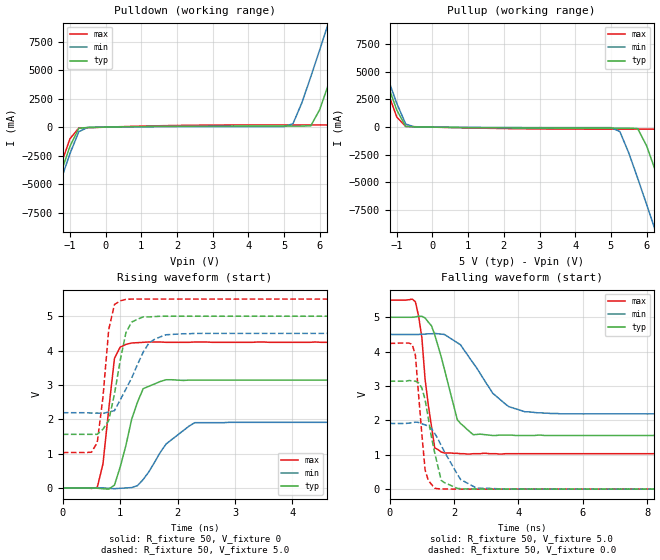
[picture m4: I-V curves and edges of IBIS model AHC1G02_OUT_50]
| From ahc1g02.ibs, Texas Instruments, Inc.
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|   Model AHC1G02_OUT_50
[Model]   AHC1G02_OUT_50
Model_type  Output
Polarity   Inverting
Vmeas = 2.50v
Cref = 15pf
| variable   typ   min   max
C_comp   3.12pf   2.34pf   3.90pf
[Temperature Range]   25   85   -40
[Voltage Range]   5.0   4.5   5.5
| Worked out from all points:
|   slope of the pulldown table from 0 to 0.75 V, typ, clamps not added: 18.8 ohm
|   slope of the pullup table from 0 to 0.75 V, typ, clamps not added: 25.3 ohm
|   rising waveform, R_fixture 50, V_fixture 0: 20-80 % time 302ps typ, 530ps min, 165ps max; typ from 0 V to 3.14 V
|   falling waveform, R_fixture 50, V_fixture 5.0: 20-80 % time 583ps typ, 1.06ns min, 315ps max; typ from 5 V to 1.56 V
|   rising waveform, R_fixture 50, V_fixture 5.0: 20-80 % time 237ps typ, 404ps min, 154ps max; typ from 1.56 V to 5 V
|   falling waveform, R_fixture 50, V_fixture 0.0: 20-80 % time 389ps typ, 678ps min, 229ps max; typ from 3.14 V to 0 V
[Pulldown]
|   Voltage   I(typ)   I(min)   I(max)
-5V       -40.9A     -41.4A     -40.3A
-1.75V    -8.76A     -9.39A     -8.09A
-1V       -1.69A     -2.33A     -1.02A
-750mV    -95.5mA    -395mA     -80.6mA
5.25V     93.4mA     298mA      192mA
5.75V     116mA      4.42A      192mA
6.25V     3.8A       9.19A      193mA
6.5V      6.17A      11.6A      931mA
6.75V     8.59A      14.1A      3.15A
7.25V     13.5A      19A        7.96A
7.5V      15.9A      21.4A      10.4A
10V       40.7A      46.2A      35.2A
[Pullup]
|   Voltage   I(typ)   I(min)   I(max)
-5V       40.7A      41.2A      40.1A
-2V       11A        11.6A      10.4A
-1.75V    8.59A      9.19A      7.96A
-1V       1.54A      2.14A      907mA
-750mV    63.6mA     284mA      62.5mA
5.25V     -84.4mA    -401mA     -178mA
5.75V     -130mA     -4.62A     -178mA
6.25V     -3.97A     -9.39A     -187mA
6.75V     -8.76A     -14.3A     -3.28A
7.25V     -13.6A     -19.2A     -8.09A
7.5V      -16.1A     -21.6A     -10.5A
10V       -40.9A     -46.4A     -35.3A
[Ramp]
| variable   typ   min   max
dV/dt_r   1.90E+00/2.83E-10   1.18E+00/5.03E-10   2.56E+00/1.41E-10
dV/dt_f   2.09E+00/5.31E-10   1.41E+00/1.01E-09   2.71E+00/2.68E-10
R_load = 50
[Rising Waveform]
R_fixture = 50
V_fixture = 0
|   Time   V(typ)   V(min)   V(max)
0s        0V         0V         0V
600ps     -9.88mV    1.95mV     11.3mV
700ps     -24.3mV    2.43uV     699mV
900ps     81.1mV     -22.5mV    3.77V
1ns       607mV      -11.8mV    4.1V
1.2ns     2V         9.68mV     4.22V
1.4ns     2.89V      243mV      4.24V
1.8ns     3.15V      1.28V      4.24V
2.3ns     3.14V      1.9V       4.25V
25ns      3.14V      1.91V      4.24V
[Falling Waveform]
R_fixture = 50
V_fixture = 5.0
V_fixture_min = 4.5
V_fixture_max = 5.5
|   Time   V(typ)   V(min)   V(max)
0s        5V         4.5V       5.5V
800ps     5.01V      4.5V       5.45V
1ns       5.03V      4.51V      4.41V
1.1ns     4.98V      4.51V      3.2V
1.4ns     4.49V      4.53V      1.2V
1.7ns     3.49V      4.5V       1.05V
2.1ns     2.02V      4.26V      1.04V
2.6ns     1.58V      3.66V      1.03V
4.2ns     1.56V      2.25V      1.03V
25ns      1.56V      2.19V      1.03V
[Rising Waveform]
R_fixture = 50
V_fixture = 5.0
V_fixture_min = 4.5
V_fixture_max = 5.5
|   Time   V(typ)   V(min)   V(max)
0s        1.56V      2.19V      1.03V
500ps     1.56V      2.18V      1.04V
600ps     1.56V      2.18V      1.32V
700ps     1.71V      2.17V      2.64V
800ps     1.96V      2.21V      4.61V
900ps     2.73V      2.25V      5.34V
1.1ns     4.52V      2.88V      5.49V
1.5ns     4.98V      4.22V      5.5V
2.1ns     5V         4.49V      5.5V
25ns      5V         4.5V       5.5V
[Falling Waveform]
R_fixture = 50
V_fixture = 0.0
|   Time   V(typ)   V(min)   V(max)
0s        3.14V      1.91V      4.24V
700ps     3.15V      1.93V      4.21V
800ps     3.14V      1.95V      3.89V
1ns       2.94V      1.9V       1.6V
1.1ns     2.61V      1.87V      559mV
1.4ns     1.05V      1.62V      24mV
1.6ns     255mV      1.27V      3.75mV
2.2ns     10.5mV     282mV      -408uV
2.7ns     2.99mV     30.1mV     412uV
25ns      0V         0V         0V
